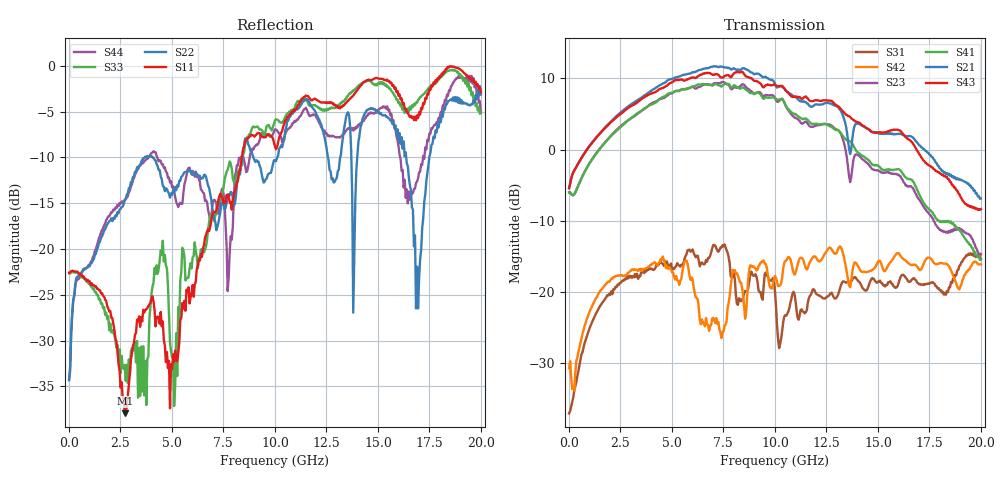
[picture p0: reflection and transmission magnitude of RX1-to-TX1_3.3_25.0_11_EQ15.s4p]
!Agilent Technologies,N5225A,MY51451112,A.09.50.13
!Agilent N5225A: A.09.50.13
!Date: Wednesday, January 31, 2018 11:06:15
!Correction: S11(Full 4 Port(1,2,3,4))
!S12(Full 4 Port(1,2,3,4))
!S13(Full 4 Port(1,2,3,4))
!S14(Full 4 Port(1,2,3,4))
!S21(Full 4 Port(1,2,3,4))
!S22(Full 4 Port(1,2,3,4))
!S23(Full 4 Port(1,2,3,4))
!S24(Full 4 Port(1,2,3,4))
!S31(Full 4 Port(1,2,3,4))
!S32(Full 4 Port(1,2,3,4))
!S33(Full 4 Port(1,2,3,4))
!S34(Full 4 Port(1,2,3,4))
!S41(Full 4 Port(1,2,3,4))
!S42(Full 4 Port(1,2,3,4))
!S43(Full 4 Port(1,2,3,4))
!S44(Full 4 Port(1,2,3,4))
!S4P File: Measurements: <S11,S12,S13,S14>,
!<S21,S22,S23,S24>,
!<S31,S32,S33,S34>,
!<S41,S42,S43,S44>:
# Hz S  RI  R 50
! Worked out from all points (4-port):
!   401 points, 10 MHz to 20 GHz, reference 50 ohm
!   strongest paths, dB at 10 MHz, 5.008 GHz, 10.01 GHz, 15 GHz, 20 GHz:
!     S43: -5.5, 9.5, 9.2, 2.4, -8.4
!     S21: -5.4, 9.9, 9.2, 2.4, -6.9
!     S41: -6.1, 8.0, 7.2, -2.2, -15.6
!     S23: -6.1, 7.9, 7.3, -2.9, -15.4
!     S42: -30.8, -17.3, -17.8, -15.8, -16.1
!     S31: -37.1, -17.0, -20.0, -18.6, -14.7
!   lowest |S11| = -37.9 dB at 2.709 GHz (marker M1), VSWR 1.03, Z = 49.1 - j0.876 ohm
!   |S11| at or under -10 dB: start of sweep to 8.398 GHz
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1e7  -0.0742 -0.00292  -0.000398 0.000568  0.014 0.000475  -0.000308 0.00037
     0.5359 0.0151  -0.0131 0.014  -0.498 -0.00306  0.0263 0.0123
     0.0139 0.00061  -0.000228 0.000487  -0.0735 -0.00409  2.9e-05 0.000516
     -0.4979 -0.00288  0.0261 0.0125  0.5333 0.0139  -0.0131 0.0145
2.70865e9  -0.009 -0.00892  0.0158 0.00341  0.0518 0.1112  0.0175 0.000716
           1.608 -1.058  0.1831 0.0166  -1.243 0.913  0.1009 0.092
           0.0591 0.1078  0.0189 0.00399  0.00477 0.0228  0.021 0.000791
           -1.096 1.061  0.0875 0.0952  1.316 -1.34  0.1824 -0.0333
6.90655e9  -0.0447 0.1339  0.0123 -0.0161  0.1367 0.063  0.00873 -0.0247
           -3.799 0.3402  0.0959 -0.1612  2.746 -0.7334  0.022 0.0159
           0.1402 0.1261  0.0169 -0.014  0.0167 0.1545  0.0205 -0.0248
           2.216 -1.778  0.0575 -0.00802  -2.786 1.951  0.0563 -0.1381
8.555725e9  -0.0117 0.3885  -0.00329 -0.0102  0.0659 0.0234  -0.00278 -0.0154
            -0.7708 3.61  -0.1466 0.3737  0.0812 -2.799  -0.0213 0.1247
            0.0898 0.0461  0.00763 -0.0126  0.0146 0.3714  -0.00132 -0.033
            -1.135 -2.407  0.00243 0.0644  1.162 3.103  0.2223 0.1785
1.04048e10  0.1358 0.448  -0.0225 -0.0475  0.00227 -0.00771  -0.0542 -0.0239
            2.378 1.324  0.2726 0.2683  -2.134 -0.6069  0.0176 0.1672
            -0.055 0.0268  -0.0297 -0.046  0.234 0.4404  -0.0593 -0.0294
            -2.13 0.5945  0.0611 0.1326  2.735 -0.2432  0.3798 -0.0992
1.415292e10  0.663 0.4092  -0.0283 -0.00312  0.0114 0.0986  -0.0127 0.0128
             0.2221 -1.481  0.436 0.1481  0.1729 0.8665  0.1537 0.0411
             0.0249 0.1108  -0.0143 -0.00121  0.752 0.252  -0.022 0.0146
             0.8282 0.4069  0.1276 0.0589  -1.264 -0.841  -0.134 -0.4677
2e10  0.7121 0.0733  0.023 0.0348  -0.0807 0.1573  0.035 0.0207
      0.0729 0.4459  0.6932 0.0744  -0.0409 -0.1654  0.1552 0.0389
      -0.0785 0.1662  0.00632 0.0479  0.5631 -0.0223  0.0476 0.0206
      -0.1662 -0.0148  0.149 0.0457  0.3723 0.0772  -0.151 -0.531
